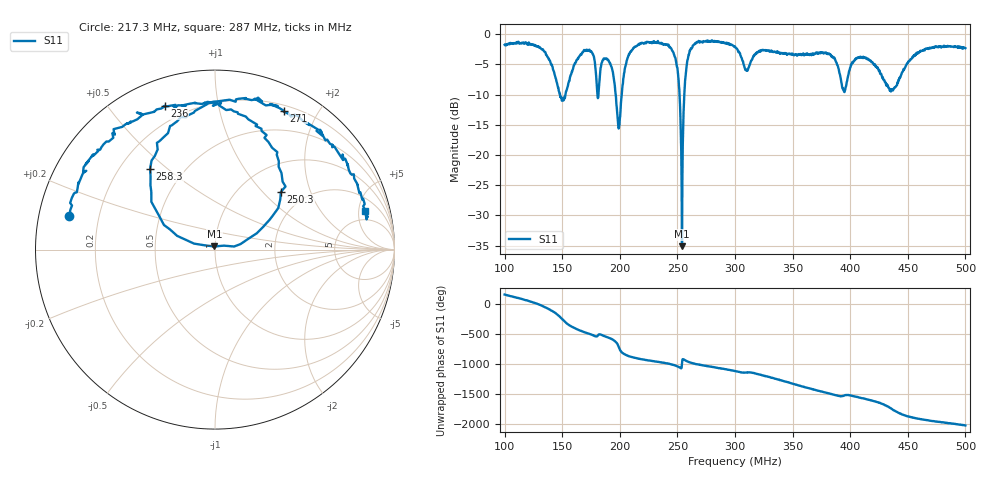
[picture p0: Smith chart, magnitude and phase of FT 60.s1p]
#  HZ  S  RI  R  50.0
! Rohde & Schwarz ZVL
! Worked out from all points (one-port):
!   1201 points, 100 MHz to 500 MHz, reference 50 ohm
!   lowest |S11| = -35.1 dB at 254 MHz (marker M1), VSWR 1.04, Z = 49.7 + j1.72 ohm
!   |S11| at or under -10 dB: 148.1 MHz to 152.8 MHz (4.689 MHz wide, 3.12 % of centre); 196.4 MHz to 201.7 MHz (5.248 MHz wide, 2.64 % of centre); 251.9 MHz to 256 MHz (4.143 MHz wide, 1.63 % of centre)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
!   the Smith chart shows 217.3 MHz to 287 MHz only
!   S11 on the Smith chart (normalised r, x): 217.3 MHz: 0.09, +0.11; 236 MHz: 0.12, +0.70; 250.3 MHz: 1.51, +1.28; 258.3 MHz: 0.32, +0.44; 271 MHz: 0.26, +1.58; 287 MHz: 3.42, +5.84
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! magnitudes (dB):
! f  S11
! 100 MHz  -1.7
! 133.3 MHz  -2.6
! 150 MHz  -10.9
! 173 MHz  -2.7
! 181 MHz  -10.6
! 191 MHz  -4.6
! 200 MHz  -14.0
! 206.3 MHz  -4.2
! 217.3 MHz  -1.5
! 236 MHz  -1.4
! 250 MHz  -5.6
! 250.3 MHz  -6.2
! 252.3 MHz  -12.0
! 254 MHz  -35.1
! 258.3 MHz  -4.8
! 271 MHz  -1.3
! 287 MHz  -1.3
! 300 MHz  -2.0
! 310 MHz  -6.1
! 322.7 MHz  -2.6
! 350 MHz  -3.2
! 383 MHz  -3.4
! 394.7 MHz  -9.5
! 400 MHz  -5.5
! 414 MHz  -4.0
! 436 MHz  -9.3
! 450 MHz  -4.8
! 500 MHz  -2.3
